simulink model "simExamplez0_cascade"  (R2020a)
settings: Solver=ode15s  StartTime=0.0  StopTime=tsim  RelTol=1e-3
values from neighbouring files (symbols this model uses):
  df = 0    [runZ0.m]
  Kc = 4/taui    (= 1)    [Recycle_example.m]    (also in runZ0.m = -0.666666666667; Main.m = 1/k*tau/(tauC+theta); runTransf.m = 1/kM(i)*tau(i)/(tauCM(i)+theta(i)); runTransfOL.m = 1/kM(i)*tau(i)/(tauCM(i)+theta(i)))
  KI = Kc/tauI    (= -0.0277777777778)    [runZ0.m]    (also in Main.m = Kp/tauIv; Main_OL.m = 1; runTransf.m = 1/kS(i)*1/tauCS(i); runTransfOL.m = 1/kS(i)*1/tauCS(i))
  td = 1    [runZ0.m]
  tv = 1    [runZ0.m]
  vf = 1    [runZ0.m]    (also in Main.m = v0+dThsp; runTransfOL.m = v00)
undefined symbols (not defined in the file or in its folder): calcv, sysDAE

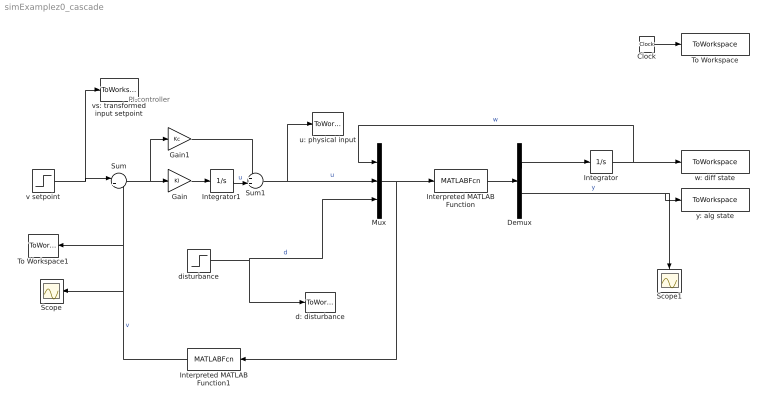
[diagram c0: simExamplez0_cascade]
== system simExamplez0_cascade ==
  note: PI-controller
  Clock : Clock
  Demux : Demux  Outputs=2
  Gain : Gain  Gain=KI  Multiplication=Matrix(K*u)
  Gain1 : Gain  Gain=Kc  Multiplication=Matrix(K*u)
  Integrator : Integrator  ZeroCross=off
  Integrator1 : Integrator
  Interpreted MATLAB Function : MATLABFcn  MATLABFcn=sysDAE(u(1),u(2),u(3))  OutputDimensions=2
  Interpreted MATLAB Function1 : MATLABFcn  MATLABFcn=calcv(u(1),u(2),u(3))  OutputDimensions=1
  Mux : Mux  Inputs=3
  Scope : Scope
  Scope1 : Scope
  Sum : Sum  Inputs=|+-
  Sum1 : Sum  Inputs=++|
  To Workspace : ToWorkspace  VariableName=timec  SampleTime=-1
  To Workspace1 : ToWorkspace  VariableName=vc  SampleTime=-1
  d: disturbance : ToWorkspace  VariableName=dc  SampleTime=-1
  disturbance : Step  Time=td  After=df  SampleTime=0
  u: physical input : ToWorkspace  VariableName=uc  SampleTime=-1
  v setpoint : Step  Time=tv  After=vf  SampleTime=0
  vs: transformed input setpoint : ToWorkspace  VariableName=vsc  SampleTime=-1
  w: diff state : ToWorkspace  VariableName=wc  SampleTime=-1
  y: alg state : ToWorkspace  VariableName=yc  SampleTime=-1
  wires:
  Interpreted MATLAB Function/1 -> Demux/1
  Demux/1 -> Integrator/1
  Integrator/1 -> Mux/1, w: diff state/1  "w"
  Demux/2 -> Scope1/1, y: alg state/1  "y"
  Mux/1 -> Interpreted MATLAB Function1/1, Interpreted MATLAB Function/1
  disturbance/1 -> d: disturbance/1, Mux/3  "d"
  v setpoint/1 -> Sum/1, vs: transformed input setpoint/1
  Clock/1 -> To Workspace/1
  Sum/1 -> Gain1/1, Gain/1
  Gain/1 -> Integrator1/1
  Interpreted MATLAB Function1/1 -> To Workspace1/1, Sum/2, Scope/1  "v"
  Sum1/1 -> u: physical input/1, Mux/2  "u"
  Integrator1/1 -> Sum1/2  "u"
  Gain1/1 -> Sum1/1
